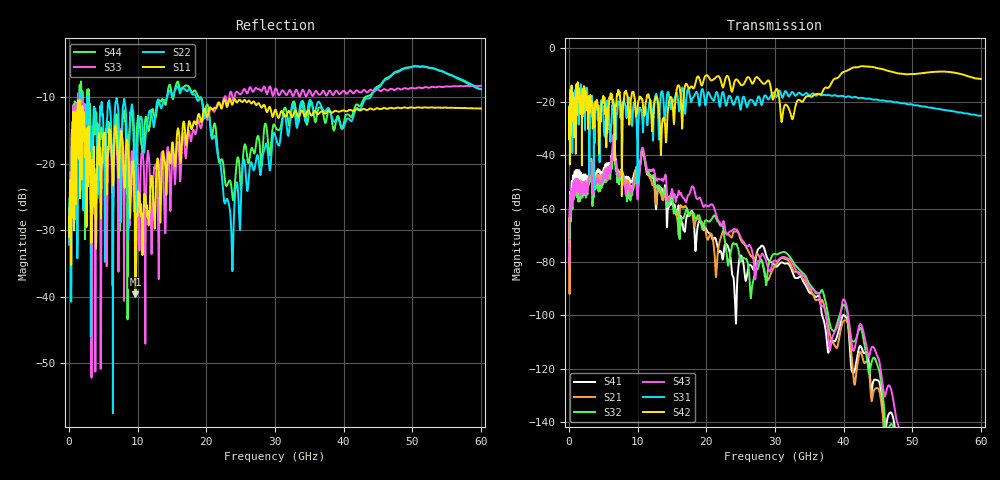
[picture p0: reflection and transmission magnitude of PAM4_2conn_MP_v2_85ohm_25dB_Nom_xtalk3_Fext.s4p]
! Info: Touchstone file created by Circ.  Input file=FAB50GbE_2conn_Midplane_Examax_Topo2_v2_85ohm_25dB_Nom.circ
# Hz S RI R 50
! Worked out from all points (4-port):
!   6000 points, 10 MHz to 60 GHz, reference 50 ohm
!   strongest paths, dB at 10 MHz, 15.01 GHz, 30.01 GHz, 45.01 GHz, 60 GHz:
!     S42: -34.0, -19.7, -16.3, -7.5, -11.4
!     S31: -33.9, -19.9, -17.5, -19.3, -25.2
!     S43: -80.7, -52.7, -79.4, -115.8, -173.2
!     S32: -67.4, -54.4, -77.0, -119.2, -166.9
!     S21: -63.7, -56.3, -81.4, -127.3, -173.6
!     S41: -66.9, -57.4, -81.4, -124.4, -190.9
!   lowest |S11| = -39.7 dB at 9.67 GHz (marker M1), VSWR 1.02, Z = 50.5 + j0.89 ohm
!   |S11| at or under -10 dB: start of sweep to end of sweep
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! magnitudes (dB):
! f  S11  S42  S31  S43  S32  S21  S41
! 10 MHz  -31.0  -34.0  -33.9  -80.7  -67.4  -63.7  -66.9
! 810 MHz  -13.3  -25.8  -17.4  -49.1  -53.9  -50.3  -46.2
! 6.43 GHz  -23.3  -19.3  -22.5  -33.4  -36.6  -35.6  -33.7
! 9.67 GHz  -39.7  -22.5  -22.0  -49.1  -48.7  -46.1  -45.6
! 21.43 GHz  -11.7  -10.8  -16.5  -62.3  -63.7  -85.4  -72.0
! 27.19 GHz  -11.2  -11.0  -21.2  -85.1  -82.7  -77.8  -78.9
! 60 GHz  -11.7  -11.4  -25.2  -173.2  -166.9  -173.6  -190.9
